FUNCTION FC 38 : VOID
TITLE =ACP_600 CONVERTER ABB
VERSION : 0.1

BEGIN
NETWORK
TITLE =START TRASFERIMENTO PARAMETRI ACP600
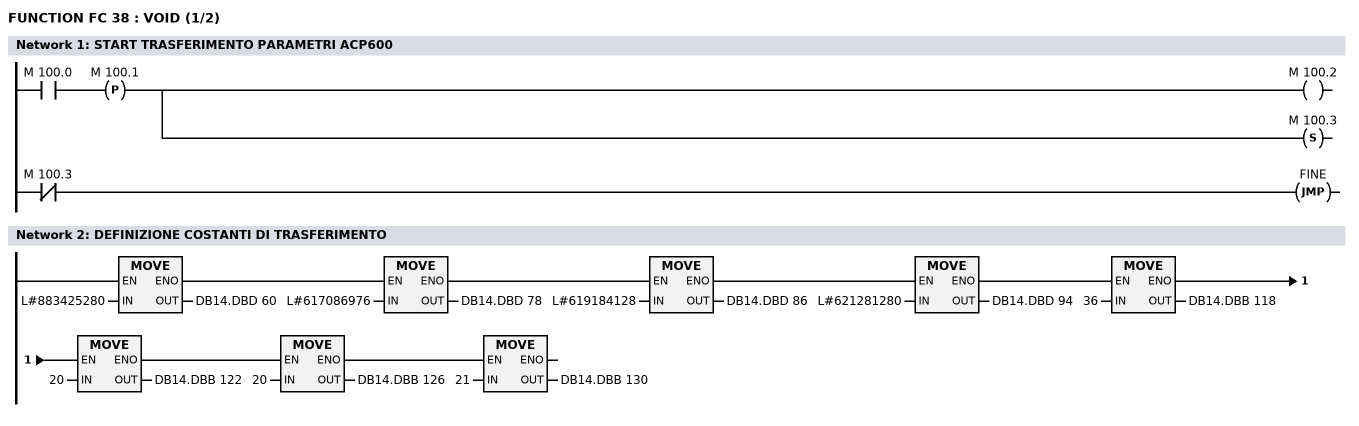
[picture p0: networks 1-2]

      U     M    100.0;
      FP    M    100.1;
      =     M    100.2;
      S     M    100.3;

      UN    M    100.3;
      SPB   FINE;


NETWORK
TITLE =DEFINIZIONE COSTANTI DI TRASFERIMENTO

      L     L#883425280;
      T     DB14.DBD   60;
      L     L#617086976;
      T     DB14.DBD   78;
      L     L#619184128;
      T     DB14.DBD   86;
      L     L#621281280;
      T     DB14.DBD   94;
      L     36;
      T     DB14.DBB  118;
      L     20;
      T     DB14.DBB  122;
      L     20;
      T     DB14.DBB  126;
      L     21;
      T     DB14.DBB  130;

NETWORK
TITLE =GESTIONE STEPS TRASFERIMENTO PARAMETRI ACP600
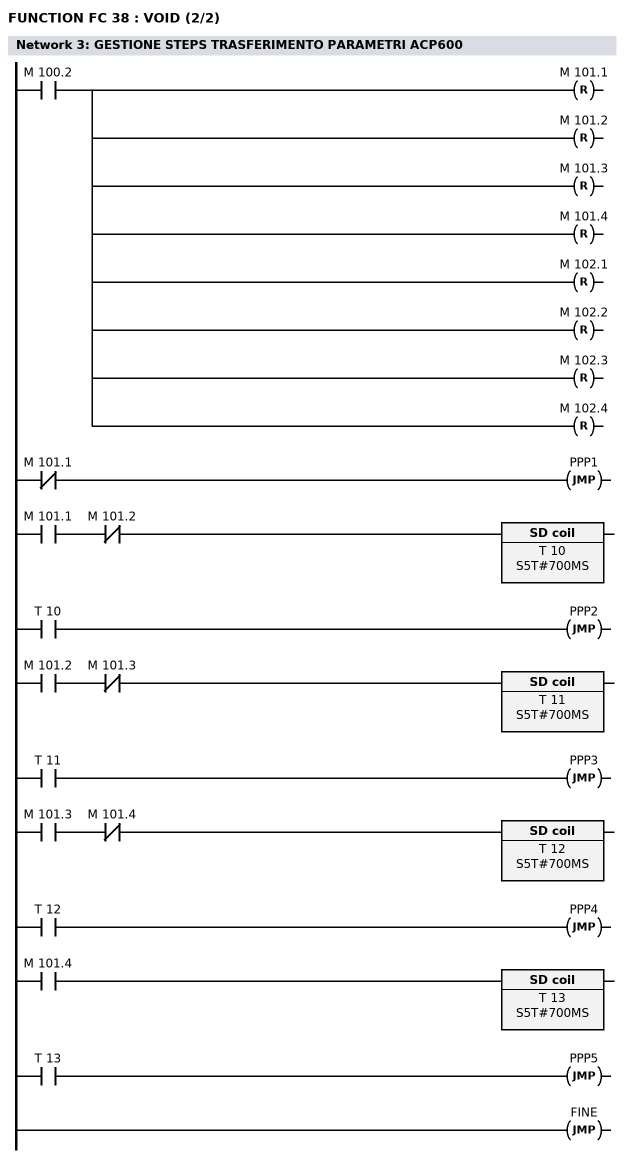
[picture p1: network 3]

      U     M    100.2;
      R     M    101.1;
      R     M    101.2;
      R     M    101.3;
      R     M    101.4;
      R     M    102.1;
      R     M    102.2;
      R     M    102.3;
      R     M    102.4;

      UN    M    101.1;
      SPB   PPP1;

      U     M    101.1;
      UN    M    101.2;
      L     S5T#700MS;
      SE    T     10;
      U     T     10;
      SPB   PPP2;

      U     M    101.2;
      UN    M    101.3;
      L     S5T#700MS;
      SE    T     11;
      U     T     11;
      SPB   PPP3;

      U     M    101.3;
      UN    M    101.4;
      L     S5T#700MS;
      SE    T     12;
      U     T     12;
      SPB   PPP4;

      U     M    101.4;
      L     S5T#700MS;
      SE    T     13;
      U     T     13;
      SPB   PPP5;
      SPA   FINE;

NETWORK
TITLE =PARAMETRO POSIZIONE

PPP1: L     DB14.DBD  134;
      L     L#52887;
      *D    ;
      L     1000;
      /D    ;
      T     DB14.DBD   64;

      CALL SFC   15 (
           LADDR                    := W#16#100,
           RECORD                   := P#DB14.DBX 60.0 BYTE 8,
           RET_VAL                  := DB14.DBW   68);

      CALL SFC   14 (
           LADDR                    := W#16#100,
           RET_VAL                  := DB14.DBW   68,
           RECORD                   := P#DB14.DBX 70.0 BYTE 8);

      S     M    101.1;
      SPA   FINE;

NETWORK
TITLE =PARAMETRO VELOCITA

PPP2: L     DB14.DBD   70;
      T     DB14.DBD  114;

      L     DB14.DBD  138;
      L     21384;
      *D    ;
      L     10000;
      /D    ;
      T     DB14.DBD   82;

      CALL SFC   15 (
           LADDR                    := W#16#100,
           RECORD                   := P#DB14.DBX 78.0 BYTE 8,
           RET_VAL                  := DB14.DBW   68);

      CALL SFC   14 (
           LADDR                    := W#16#100,
           RET_VAL                  := DB14.DBW   68,
           RECORD                   := P#DB14.DBX 70.0 BYTE 8);

      S     M    101.2;
      SPA   FINE;

NETWORK
TITLE =PARAMETRO ACCELERAZIONE
//VALORE A PANNELLO IN PERCENTUALE
PPP3: L     DB14.DBD   70;
      T     DB14.DBD  102;

      L     DB14.DBD  282;
      L     2;
      *D    ;
      T     DB14.DBD   90;


      CALL SFC   15 (
           LADDR                    := W#16#100,
           RECORD                   := P#DB14.DBX 86.0 BYTE 8,
           RET_VAL                  := DB14.DBW   68);

      CALL SFC   14 (
           LADDR                    := W#16#100,
           RET_VAL                  := DB14.DBW   68,
           RECORD                   := P#DB14.DBX 70.0 BYTE 8);

      S     M    101.3;
      SPA   FINE;

NETWORK
TITLE =PARAMETRO DECELERAZIONE
//IL VALORE A PANNELLO IN PERCENTUALE
PPP4: L     DB14.DBD   70;
      T     DB14.DBD  106;

      L     DB14.DBD  142;
      L     -2;
      *D    ;
      T     DB14.DBD   98;
//
      CALL SFC   15 (
           LADDR                    := W#16#100,
           RECORD                   := P#DB14.DBX 94.0 BYTE 8,
           RET_VAL                  := DB14.DBW   68);

      CALL SFC   14 (
           LADDR                    := W#16#100,
           RET_VAL                  := DB14.DBW   68,
           RECORD                   := P#DB14.DBX 70.0 BYTE 8);

      S     M    101.4;
      SPA   FINE;

PPP5: L     DB14.DBD   70;
      T     DB14.DBD  110;

      CALL SFC   14 (
           LADDR                    := W#16#100,
           RET_VAL                  := DB14.DBW   68,
           RECORD                   := P#DB14.DBX 70.0 BYTE 8);

      L     DB14.DBD   70;
      T     DB14.DBD  114;

NETWORK
TITLE =VERIFICA COMUNICAZIONE OK
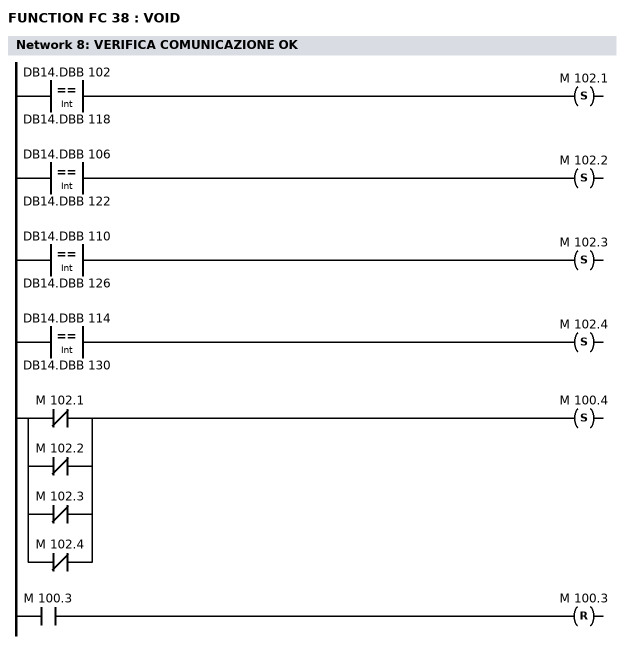
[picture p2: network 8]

      L     DB14.DBB  102;
      L     DB14.DBB  118;
      ==I   ;
      S     M    102.1;

      L     DB14.DBB  106;
      L     DB14.DBB  122;
      ==I   ;
      S     M    102.2;

      L     DB14.DBB  110;
      L     DB14.DBB  126;
      ==I   ;
      S     M    102.3;

      L     DB14.DBB  114;
      L     DB14.DBB  130;
      ==I   ;
      S     M    102.4;

      U(    ;
      ON    M    102.1;
      ON    M    102.2;
      ON    M    102.3;
      ON    M    102.4;
      )     ;
      S     M    100.4;

      U     M    100.3;
      R     M    100.3;

NETWORK
TITLE =FINE TRASMISSIONE

FINE: NOP   0;

END_FUNCTION

